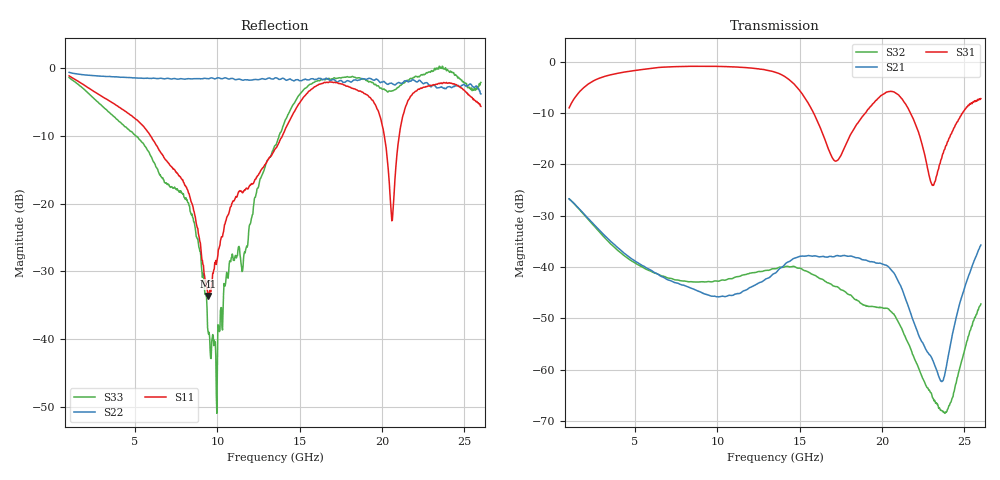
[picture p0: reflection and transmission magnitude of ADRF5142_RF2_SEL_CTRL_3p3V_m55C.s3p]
! Device: ADRF5142
! Description: Silicon, SPDT Switch, Reflective
! Frequency: 8.00 GHz - 11.00 GHz
! Ports:
!  RFC = Port 1
!  RF1 = Port 2
!  RF2 = Port 3
! VDD = +3.3V
! VSS = -3.3V
! CTRL = +3.3V
! Temp = -55C
! Data:  Data was collected using an calibrated 4 port network analyzer.
!  The reference plane is the package pins of ADRF5142 switch.
! Notes: Analog Devices supplies this data as a sample of measured data
!  for this product.  Your particular data for this product may vary.
!  Data was taken at -55 degrees C.
!  Analog Devices reserves the right to change this data at anytime.
# HZ S DB R 50
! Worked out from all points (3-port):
!   801 points, 1 GHz to 26 GHz, reference 50 ohm
!   strongest paths, dB at 1 GHz, 7.25 GHz, 13.5 GHz, 19.75 GHz, 26 GHz:
!     S31: -9.0, -1.0, -2.0, -7.2, -7.2
!     S21: -26.7, -42.8, -41.2, -39.3, -35.7
!     S32: -26.7, -42.3, -40.3, -47.9, -47.2
!   lowest |S11| = -33.6 dB at 9.438 GHz (marker M1), VSWR 1.04, Z = 51 - j1.84 ohm
!   |S11| at or under -10 dB: 5.935 GHz to 13.95 GHz (8.017 GHz wide, 80.6 % of centre); 20.14 GHz to 21.04 GHz (907.2 MHz wide, 4.41 % of centre)
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1e9  -1.17 158.8  -26.74 -42.2  -9.01 38.8
     -26.74 -42.2  -0.66 169.9  -26.74 -61.4
     -9.01 38.8  -26.74 -61.4  -1.43 122.4
2.8437e9  -3.99 131.9  -32.82 -87.9  -3.23 -16.8
          -32.82 -87.9  -1.22 154.4  -33.16 -142.8
          -3.23 -16.8  -33.16 -142.8  -5.28 32.0
5.875e9  -9.74 95.6  -40.45 -114.5  -1.36 -90.0
         -40.45 -114.5  -1.55 132.3  -40.71 138.4
         -1.36 -90.0  -40.71 138.4  -12.55 -81.9
9.4375e9  -33.60 -59.5  -45.44 -129.0  -0.91 -172.6
          -45.44 -129.0  -1.62 102.0  -42.82 63.7
          -0.91 -172.6  -42.82 63.7  -38.90 -112.1
1.35e10  -11.96 -106.3  -41.20 -140.7  -2.05 81.9
         -41.20 -140.7  -1.47 70.2  -40.31 -36.5
         -2.05 81.9  -40.31 -36.5  -11.46 43.4
1.71562e10  -2.14 170.6  -37.89 138.9  -19.36 34.6
            -37.89 138.9  -1.87 44.9  -43.79 -163.2
            -19.36 34.6  -43.79 -163.2  -1.53 -98.4
2.05937e10  -22.54 -27.4  -40.70 49.1  -5.82 -7.8
            -40.70 49.1  -2.28 13.1  -48.79 63.3
            -5.82 -7.8  -48.79 63.3  -3.39 -163.6
2.20625e10  -3.42 170.5  -51.83 27.8  -12.50 -70.7
            -51.83 27.8  -2.03 0.5  -58.48 -8.7
            -12.50 -70.7  -58.48 -8.7  -1.25 179.7
2.3625e10  -2.30 95.4  -62.31 116.8  -18.77 4.4
           -62.31 116.8  -2.86 -16.6  -67.96 -72.1
           -18.77 4.4  -67.96 -72.1  -0.06 144.9
2.6e10  -5.67 6.7  -35.72 162.9  -7.22 -49.2
        -35.72 162.9  -3.84 -28.1  -47.19 133.2
        -7.22 -49.2  -47.19 133.2  -2.14 84.8
